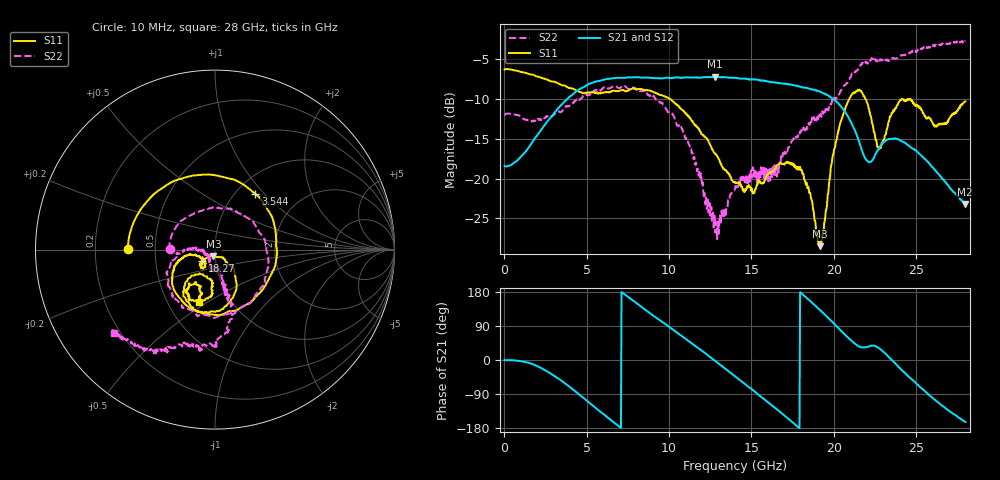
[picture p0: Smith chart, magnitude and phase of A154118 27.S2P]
!  2-Port S-parameters saved by WinCal
! VAR MeasName=S-Parameters (CALIBRATED_DATA) read from VNA (N5230A)
! VAR MeasDate=2015-9-10 14:36:25
! VAR NAME=A154118 27
! VAR FILENAME=A154118 27.S2P
! VAR DATE=2015-9-10 14:36:25
! VAR PHYS_PORTS=1,2
# Hz S DB R 50
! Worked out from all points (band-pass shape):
!   801 points, 10 MHz to 28 GHz, reference 50 ohm
!   highest |S21| = -7.24 dB at 12.78 GHz (marker M1); lowest = -23.2 dB at 27.97 GHz (marker M2)
!   |S21| within 3 dB of the highest: 3.716 GHz to 20.1 GHz (16.39 GHz wide, 138 % of centre)
!   lowest |S11| = -28.5 dB at 19.18 GHz (marker M3), VSWR 1.08, Z = 49 - j3.6 ohm
!   |S11| at or under -10 dB: 10.02 GHz to 20.95 GHz (10.93 GHz wide, 70.5 % of centre); 21.91 GHz to end of sweep
!   |S22| runs from -27.6 to -2.7 dB; largest |S21 - S12| = 0.0077
!   S11 on the Smith chart (normalised r, x): 10 MHz: 0.35, +0.00; 3.544 GHz: 1.23, +0.89; 18.27 GHz: 0.86, -0.11; 28 GHz: 0.71, -0.46
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1e7  -6.34 179.6  -18.43 -0.0  -18.47 0.0  -12.09 179.8
1.864338e9  -7.12 117.4  -14.92 -13.7  -14.94 -13.5  -12.80 99.8
3.543738e9  -8.34 54.0  -10.59 -57.2  -10.58 -57.3  -11.44 19.5
4.698325e9  -9.24 8.3  -8.68 -96.5  -8.65 -96.8  -9.89 -28.6
6.972512e9  -9.03 -66.1  -7.40 -175.9  -7.35 -176.2  -8.67 -97.7
9.351662e9  -9.44 -123.7  -7.46 107.5  -7.41 107.3  -10.37 -151.1
1.09261e10  -11.62 -152.6  -7.35 58.4  -7.31 57.9  -14.46 -175.7
1.278044e10  -16.86 -168.2  -7.24 -1.4  -7.21 -2.1  -24.66 -140.9
1.4005e10  -20.54 -156.8  -7.42 -42.7  -7.41 -43.3  -21.29 -108.6
1.585934e10  -19.93 -125.1  -7.79 -106.7  -7.74 -107.0  -20.05 -97.2
1.827348e10  -20.39 -138.8  -8.61 167.3  -8.67 166.7  -13.54 -74.9
1.869332e10  -22.82 -136.2  -8.84 151.1  -8.87 150.5  -12.36 -76.0
1.918315e10  -28.47 -103.5  -9.12 131.3  -9.15 130.6  -12.09 -77.6
2.005784e10  -16.20 -46.1  -10.17 94.4  -10.16 94.0  -10.10 -71.8
2.10025e10  -9.87 -80.0  -12.76 53.8  -12.70 53.1  -7.33 -80.1
2.21221e10  -11.20 -128.6  -17.92 35.6  -17.93 34.4  -5.39 -94.9
2.275188e10  -16.34 -116.1  -16.16 31.3  -16.21 30.6  -5.34 -102.9
2.334666e10  -12.84 -93.3  -15.05 7.7  -15.06 7.3  -5.23 -107.5
2.516601e10  -10.89 -124.7  -16.83 -68.1  -16.86 -68.7  -3.93 -119.2
2.621564e10  -13.36 -120.6  -19.05 -107.6  -19.07 -107.6  -3.27 -125.3
2.796501e10  -10.37 -107.6  -23.20 -162.9  -23.10 -163.0  -2.78 -141.8
2.8e10  -10.34 -107.0  -23.16 -163.7  -23.19 -164.3  -2.71 -140.3
